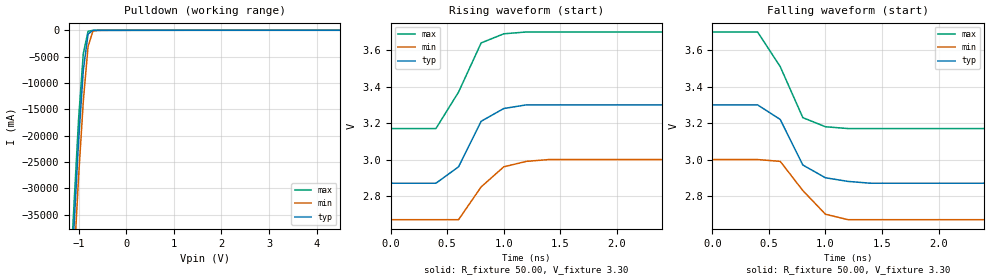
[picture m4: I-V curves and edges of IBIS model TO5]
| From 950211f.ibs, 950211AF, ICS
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|   Model TO5
[Model]   TO5
Model_type   Open_drain
Polarity   Inverting
|Vinl = 800.00mV
|Vinh =   2.00V
C_comp   5.50pF   5.00pF   6.00pF
[Temperature Range]   27.00   70.00   0.00
[Voltage Range]   3.30V   3.00V   3.70V
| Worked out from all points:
|   slope of the pulldown table from 0 to 0.495 V, typ, clamps not added: 122 ohm
|   rising waveform, R_fixture 50.00, V_fixture 3.30: 20-80 % time 220ps typ, 279ps min, 260ps max; typ from 2.87 V to 3.3 V
|   falling waveform, R_fixture 50.00, V_fixture 3.30: 20-80 % time 235ps typ, 275ps min, 256ps max; typ from 3.3 V to 2.87 V
[Pulldown]
| voltage   I(typ)   I(min)   I(max)
-3.3V     -431.7A    -437.9A    -427.9A
-1.5V     -105.8A    -112.6A    -101.5A
-1V       -21.13A    -27.91A    -16.98A
-900mV    -7.57A     -13.43A    -4.4A
-800mV    -689.4mA   -3.07A     -180.9mA
-700mV    -25mA      -186.7mA   -11.64mA
-600mV    -6.45mA    -11.8mA    -6.72mA
6.2V      12.17mA    9.78mA     14.58mA
[Ramp]
| variable   typ   min   max
dV/dt_r   255.60m/171.20p   201.00m/169.75p   319.20m/188.31p
dV/dt_f   255.60m/200.00p   201.00m/200.00p   319.20m/200.00p
[Rising Waveform]
R_fixture = 50.00
V_fixture = 3.30
V_fixture_min = 3.00
V_fixture_max = 3.70
| time   V(typ)   V(min)   V(max)
0s        2.87V      2.67V      3.17V
400ps     2.87V      2.67V      3.17V
600ps     2.96V      2.67V      3.37V
800ps     3.21V      2.85V      3.64V
1ns       3.28V      2.96V      3.69V
1.2ns     3.3V       2.99V      3.7V
1.4ns     3.3V       3V         3.7V
10ns      3.3V       3V         3.7V
[Falling Waveform]
R_fixture = 50.00
V_fixture = 3.30
V_fixture_min = 3.00
V_fixture_max = 3.70
| time   V(typ)   V(min)   V(max)
0s        3.3V       3V         3.7V
400ps     3.3V       3V         3.7V
600ps     3.22V      2.99V      3.51V
800ps     2.97V      2.83V      3.23V
1ns       2.9V       2.7V       3.18V
1.2ns     2.88V      2.67V      3.17V
1.4ns     2.87V      2.67V      3.17V
10ns      2.87V      2.67V      3.17V
